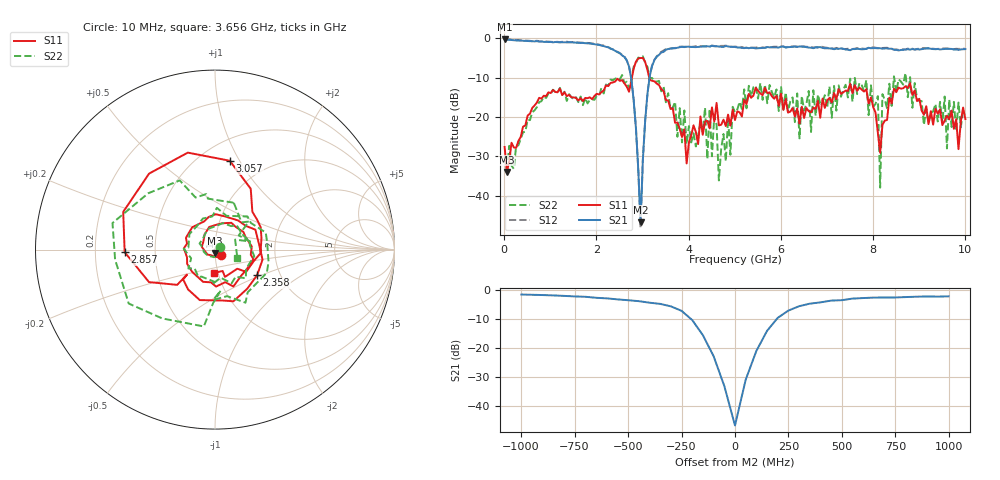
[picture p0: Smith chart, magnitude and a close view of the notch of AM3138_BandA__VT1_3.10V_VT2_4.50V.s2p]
! Date/Time: Tue, Nov 13, 2018 4:42 PM
! Network Analyzer: Agilent Technologies E8364B Rev: A.07.50.67
! Sweep from 0.010 to 10.000 GHz, 201 Points, Sweep Type: LIN
! Power Supply: 3.101 V, 0.000 A
# Hz S DB R 50
!freq MagS11 AngS11 MagS21 AngS21 MagS12 AngS12 MagS22 AngS22
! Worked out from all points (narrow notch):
!   201 points, 10 MHz to 10 GHz, reference 50 ohm
!   highest |S21| = -0.28 dB at 10 MHz (marker M1); lowest = -46.8 dB at 2.957 GHz (marker M2)
!   notch at M2: 44.3 dB deep, 173 MHz wide at half that depth
!   lowest |S11| = -33.9 dB at 59.95 MHz (marker M3), VSWR 1.04, Z = 49.8 - j2 ohm
!   |S11| at or under -10 dB: start of sweep to 2.77 GHz; 3.145 GHz to end of sweep
!   |S22| runs from -37.9 to -4.6 dB; largest |S21 - S12| = 0.03
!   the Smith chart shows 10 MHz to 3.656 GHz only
!   S11 on the Smith chart (normalised r, x): 10 MHz: 1.06, -0.06; 2.358 GHz: 1.53, -0.47; 2.857 GHz: 0.33, -0.01; 3.057 GHz: 0.69, +0.91; 3.656 GHz: 0.96, -0.25
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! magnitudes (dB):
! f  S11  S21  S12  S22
! 10 MHz  -27.6  -0.3  -0.2  -30.1
! 59.95 MHz  -33.9  -0.4  -0.3  -33.1
! 759.2 MHz  -15.1  -0.9  -0.8  -16.2
! 1.708 GHz  -16.0  -1.2  -1.1  -17.0
! 2.358 GHz  -11.2  -2.9  -2.8  -10.6
! 2.857 GHz  -6.0  -22.9  -22.6  -6.3
! 2.957 GHz  -5.0  -46.8  -48.1  -5.0
! 3.057 GHz  -6.0  -21.0  -21.0  -6.3
! 3.357 GHz  -11.9  -4.2  -4.0  -10.8
! 3.656 GHz  -17.8  -2.6  -2.5  -17.5
! 3.956 GHz  -31.8  -2.2  -2.2  -26.8
! 4.555 GHz  -21.2  -2.0  -2.0  -19.8
! 4.655 GHz  -22.1  -2.1  -2.0  -36.1
! 5.005 GHz  -20.8  -2.2  -2.1  -18.8
! 6.404 GHz  -21.7  -2.1  -2.0  -25.4
! 6.703 GHz  -17.6  -2.5  -2.4  -13.2
! 7.952 GHz  -15.1  -2.6  -2.4  -12.0
! 8.102 GHz  -23.9  -2.6  -2.5  -14.7
! 8.152 GHz  -29.1  -2.5  -2.5  -37.9
! 8.202 GHz  -21.9  -2.7  -2.5  -14.2
! 8.352 GHz  -15.1  -2.7  -2.7  -11.6
! 10 GHz  -20.5  -2.8  -2.7  -18.9
